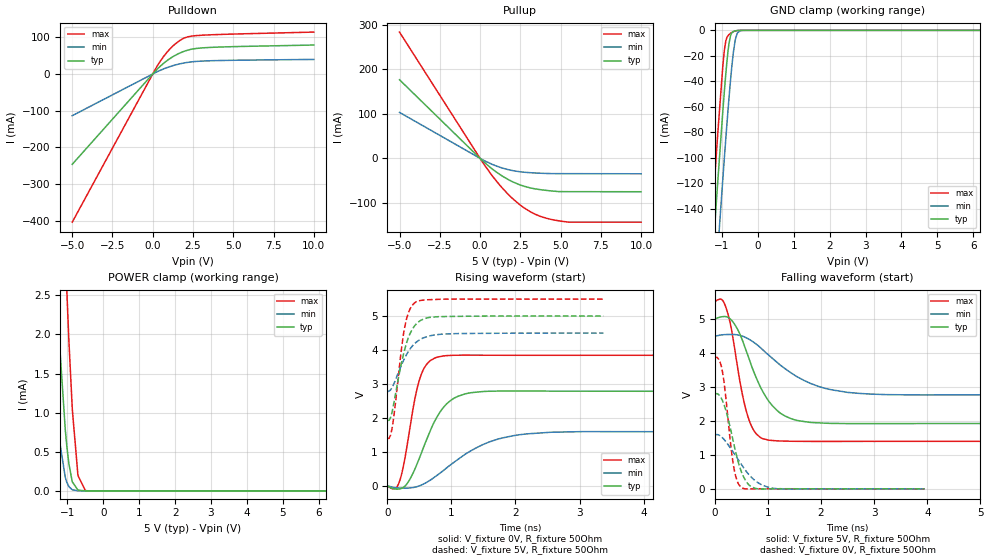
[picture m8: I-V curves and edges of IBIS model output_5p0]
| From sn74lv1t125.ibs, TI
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|   output_5p0 Model
[Model]   output_5p0
Model_type   3-state
Polarity   Non-Inverting
Vmeas = 2.5
Vref = 0
Cref = 50pF
Rref = 100
|   typ   min   max
|   (nom PVT)   (fast PVT)   (slow PVT)
C_comp   3.036e-12   2.933e-12   3.166e-12
| Where nom  PVT is Nominal Process, 5V, 40C
|   Fast PVT is Strong Process,  5.5V, -40C
|   Slow PVT is Weak Process,   4.5V, 140C
[Voltage Range]   5   4.5   5.5
|Junction Temperature
[Temperature Range]   40   140   -40
[Pullup Reference]   5   4.5   5.5
[Pulldown Reference]   0   0   0
[Power Clamp Reference]   5   4.5   5.5
[GND Clamp Reference]   0   0   0
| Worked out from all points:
|   slope of the pulldown table from 0 to 0.75 V, typ, clamps not added: 23.6 ohm
|   slope of the pullup table from 0 to 0.75 V, typ, clamps not added: 31.5 ohm
|   GND clamp passes 1 mA (typ) near -0.68 V on its own axis
|   POWER clamp passes 1 mA (typ) near -1.09 V on its own axis
|   falling waveform, V_fixture 5V, R_fixture 50Ohm: 20-80 % time 518ps typ, 916ps min, 290ps max; typ from 5 V to 1.93 V
|   rising waveform, V_fixture 0V, R_fixture 50Ohm: 20-80 % time 399ps typ, 782ps min, 224ps max; typ from 0 V to 2.79 V
|   rising waveform, V_fixture 5V, R_fixture 50Ohm: 20-80 % time 221ps typ, 281ps min, 160ps max; typ from 1.93 V to 5 V
|   falling waveform, V_fixture 0V, R_fixture 50Ohm: 20-80 % time 264ps typ, 441ps min, 164ps max; typ from 2.79 V to 0 V
[Pulldown]
|   Voltage   I(typ)   I(min)   I(max)
-5V       -246.2mA   -113.7mA   -403.9mA
263.5mV   12.5mA     5.885mA    20.71mA
795mV     33.37mA    15.92mA    54.53mA
1.242V    46.91mA    22.57mA    75.87mA
1.528V    53.84mA    26.02mA    86.51mA
1.985V    62.35mA    30.29mA    98.41mA
2.663V    69.36mA    34.08mA    104.4mA
4.295V    73.6mA     36.78mA    107.8mA
10V       78.88mA    39.67mA    114.2mA
[GND Clamp]
|   Voltage   I(typ)   I(min)   I(max)
-5V       -1.841A    -1.864A    -1.827A
-1.288V   -190.5mA   -243.9mA   -153.5mA
-1.244V   -172mA     -225.7mA   -134.7mA
-1.145V   -131.3mA   -185.2mA   -93.5mA
-1.115V   -119.1mA   -173mA     -81.25mA
-974mV    -63.74mA   -116.8mA   -28.23mA
-930mV    -47.7mA    -99.88mA   -15.61mA
-801.5mV  -10.29mA   -53.12mA   -3.37mA
-680mV    -924.7uA   -17.3mA    -1.009mA
-572mV    -177.5uA   -2.26mA    -187.4uA
-432.5mV  -14.78uA   -69.02uA   -9.767uA
10V       0A         0A         0A
[Pullup]
|   Voltage   I(typ)   I(min)   I(max)
-5V       176.7mA    103.3mA    283.9mA
314.5mV   -10.58mA   -6.152mA   -17.06mA
769.5mV   -24.34mA   -13.79mA   -39.84mA
1.367V    -39.63mA   -21.66mA   -66.27mA
1.9V      -50.61mA   -26.73mA   -86.4mA
2.425V    -59.02mA   -30.06mA   -103.1mA
3.08V     -66.23mA   -32.31mA   -119.3mA
3.696V    -70.27mA   -33.5mA    -129.9mA
4.894V    -74.87mA   -34.52mA   -140.7mA
5.503V    -75.05mA   -34.56mA   -143.7mA
10V       -75.22mA   -34.82mA   -143.7mA
[POWER Clamp]
|   Voltage   I(typ)   I(min)   I(max)
-5V       77.24mA    42.94mA    125.9mA
-1.742V   7.367mA    3.544mA    15.7mA
-1.496V   4.442mA    1.946mA    10.39mA
-1.31V    2.599mA    976.9uA    6.864mA
-1.26V    2.18mA     767.8uA    6.034mA
-1.056V   778.3uA    171.9uA    3.069mA
-1.013V   566.1uA    108.6uA    2.542mA
-955mV    340.7uA    54.1uA     1.904mA
-860mV    115.2uA    14.7uA     1.035mA
-704.5mV  10.48uA    1.48uA     198.1uA
-500mV    371nA      82.56nA    5.271uA
10V       0A         0A         0A
[Ramp]
R_load = 50
|   typ   min   max
dV/dt_r   1.67219/3.9833e-10   0.953974/7.8106e-10   2.30762/2.24062e-10
dV/dt_f   1.84348/5.17153e-10   1.03365/9.15033e-10   2.46005/2.90383e-10
[Falling Waveform]
V_fixture = 5V
V_fixture_min = 4.5V
V_fixture_max = 5.5V
R_fixture = 50Ohm
|   Time   V(typ)   V(min)   V(max)
0s        5V         4.5V       5.5V
200ps     5.079V     4.546V     5.395V
300ps     4.996V     4.549V     4.824V
400ps     4.786V     4.543V     3.884V
600ps     4.038V     4.447V     2.261V
750ps     3.394V     4.301V     1.685V
925ps     2.811V     4.068V     1.468V
1.45ns    2.061V     3.404V     1.403V
2.5ns     1.924V     2.842V     1.399V
8.575ns   1.928V     2.777V     1.4V
[Rising Waveform]
V_fixture = 0V
V_fixture_min = 0V
V_fixture_max = 0V
R_fixture = 50Ohm
|   Time   V(typ)   V(min)   V(max)
0s        690.4pV    4.014nV    1.62nV
175ps     -93.59mV   -60.08mV   62.7mV
325ps     115.7mV    -62.11mV   1.39V
500ps     820.7mV    3.087mV    3.126V
625ps     1.422V     119.1mV    3.607V
775ps     2.033V     312.1mV    3.789V
950ps     2.458V     570mV      3.838V
1.2ns     2.701V     914.3mV    3.849V
2.175ns   2.794V     1.532V     3.846V
7.275ns   2.787V     1.59V      3.846V
[Rising Waveform]
V_fixture = 5V
V_fixture_min = 4.5V
V_fixture_max = 5.5V
R_fixture = 50Ohm
|   Time   V(typ)   V(min)   V(max)
0s        1.928V     2.777V     1.4V
50ps      2.017V     2.828V     1.496V
75ps      2.192V     2.903V     1.718V
225ps     3.668V     3.586V     4.115V
275ps     4.054V     3.783V     4.722V
350ps     4.472V     4.023V     5.199V
425ps     4.713V     4.19V      5.39V
600ps     4.935V     4.382V     5.476V
875ps     4.985V     4.47V      5.496V
3.375ns   5V         4.5V       5.5V
[Falling Waveform]
V_fixture = 0V
V_fixture_min = 0V
V_fixture_max = 0V
R_fixture = 50Ohm
|   Time   V(typ)   V(min)   V(max)
0s        2.787V     1.59V      3.846V
50ps      2.804V     1.599V     3.868V
125ps     2.67V      1.538V     3.613V
175ps     2.486V     1.458V     3.158V
350ps     1.399V     1.078V     715.8mV
425ps     898.6mV    902.3mV    219mV
500ps     510.7mV    724.8mV    41.64mV
675ps     79.95mV    366.6mV    -2.439mV
1.1ns     460.9uV    15.9mV     1.555mV
3.95ns    -43.29uV   -194.6uV   9.014uV
